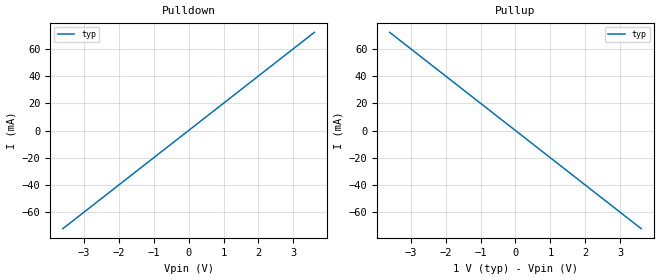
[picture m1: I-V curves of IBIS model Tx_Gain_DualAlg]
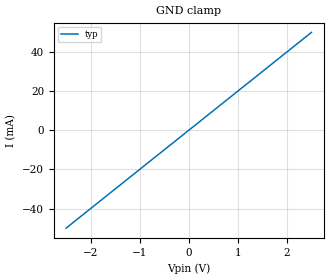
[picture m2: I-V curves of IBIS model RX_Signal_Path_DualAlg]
| DO NOT MAKE ANY EDITS IN THIS FILE. THEY CAN BE LOST WHEN THE NEXT BUILD RUNS.
[IBIS Ver] 6.0
[File Name]   TDP2004_DualAlg.ibs
[File Rev]   1.0
[Component]   TDP2004_DualAlg
[Manufacturer] Texas Instruments
[Package]
R_pkg 0.001m   NA   NA
L_pkg 0.001nH  NA   NA
C_pkg 0.001pF  NA   NA
[Pin]   signal_name  model_name   R_pin L_pin  C_pin
1P   Tx_Gain_DualAlg_P   Tx_Gain_DualAlg
1N   Tx_Gain_DualAlg_N   Tx_Gain_DualAlg
2P   RX_Signal_Path_DualAlg_2P   RX_Signal_Path_DualAlg
2N   RX_Signal_Path_DualAlg_2N   RX_Signal_Path_DualAlg
[Diff_Pin] inv_pin vdiff tdelay_typ tdelay_min tdelay_max
1P   1N   NA   NA   NA   NA
2P   2N   NA   NA   NA   NA
| Models and submodels in the file (2): Tx_Gain_DualAlg (Output), RX_Signal_Path_DualAlg (Input)
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| Tx Model
[Model] Tx_Gain_DualAlg
Model_type Output
C_comp 0.02p NA NA
Cref = 0
Vref = 0.5
Rref = 50
Vmeas = 0.5
[Algorithmic Model]
Executable Windows_cl19.29.30147_64 Tx_Gain_DualAlg_x64.dll Tx_Gain_DualAlg.ami
Executable Linux_gcc4.7.2_64 Tx_Gain_DualAlg.so Tx_Gain_DualAlg.ami
[End Algorithmic Model]
[Temperature_Range] 50 NA NA
[Voltage Range] 1 NA NA
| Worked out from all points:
|   slope of the pulldown table from 0 to 0.15 V, typ, clamps not added: 50 ohm
|   slope of the pullup table from 0 to 0.15 V, typ, clamps not added: 50 ohm
[Pulldown]
-3.6V     -72mA      NA         NA
0V        0A         NA         NA
3.6V      72mA       NA         NA
[Pullup]
-3.6V     72mA       NA         NA
0V        0A         NA         NA
3.6V      -72mA      NA         NA
[GND Clamp]
-3.6V     0A         NA         NA
0V        0A         NA         NA
3.6V      0A         NA         NA
[Power Clamp]
-3.6V     0A         NA         NA
0V        0A         NA         NA
3.6V      0A         NA         NA
[Ramp]
dV/dt_r   0.3/1.5p   NA   NA
dV/dt_f   0.3/1.5p   NA   NA
R_load  =   50
| Rx Model
[Model] RX_Signal_Path_DualAlg
Model_type Input
C_comp   0.01p   NA   NA
Vinh = 0.25
Vinl = -0.25
[Algorithmic Model]
Executable Windows_cl19.29.30147_64 RX_Signal_Path_DualAlg_x64.dll RX_Signal_Path_DualAlg.ami
Executable Linux_gcc4.7.2_64 RX_Signal_Path_DualAlg_x64.so RX_Signal_Path_DualAlg.ami
[End Algorithmic Model]
[Temperature Range]   50   NA   NA
[Voltage Range]   1   NA   NA
[GND Clamp]
-2.5V     -50mA      NA         NA
0V        0A         NA         NA
2.5V      50mA       NA         NA
